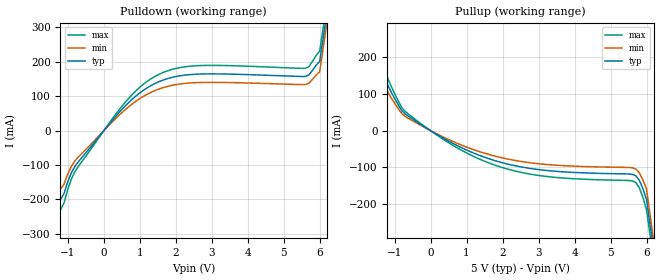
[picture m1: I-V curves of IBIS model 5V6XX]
[IBIS Ver]   2.1
[File name]   55202_5.ibs
[File Rev]   2.0
[Date]   7/20/01
[Source]   ICS MicroClock Applications Engineering 2
[Disclaimer] This information is for modeling purposes only, and is
(C) Copyright Integrated Circuit Systems, Inc. 1997-2001
   All rights reserved
ICS hereby grants the user of this IBIS model a non-exclusive,
nontransferable license to use this IBIS model under the following terms.
Before using this IBIS model, the user should read this license.
If the user does not accept these terms,  the IBIS model should be
returned to ICS within 30 days.
   The user is granted this license only to use the IBIS model and
is not granted rights to sell, load, rent, lease or license the IBIS
model in whole or in part, or in modified form to anyone other than
user. User may modify the IBIS model to suit its specific
applications but rights to derivative works and such modifications
shall belong to ICS.
   This IBIS model is provided on an "AS IS" basis and ICS makes
absolutely no warranty with respect to the information contained
herein. ICS DISCLAIMS AND CUSTOMER WAIVES ALL WARRANTIES, EXPRESS
OR IMPLIED, INCLUDING WARRANTIES OF MERCHANTABILITY OR FITNESS FOR
A PARTICULAR PURPOSE. The entire risk as to quality and performance
is with the Customer. ACCORDINGLY, IN NO EVENT SHALL THE COMPANY BE
LIABLE FOR ANY DAMAGES, WHETHER IN CONTRACT OR TORT,INCLUDING ANY
LOST PROFITS OR OTHER INCIDENTAL, CONSEQUENTIAL, EXEMPLARY, OR
PUNITIVE DAMAGES ARISING OUT OF THE USE OR APPLICATION OF THE IBIS
model provided in this package. Further, ICS reserves the right to
make changes without notice to any product herein to improve
reliability, function, or design. ICS does not convey any license
under patent rights or any other intellectual property rights,
including those of third parties.
   ICS is not obligated to provide maintenance or support
for the licensed IBIS model.
[Component]   ICS552-02
[Manufacturer] Integrated Circuit Systems Inc.
[Package]
|   typ   min   max
R_pkg   40m   35m   45m
L_pkg   1.65nH   1.35nH   1.95nH
C_pkg   0.24pF   0.14pF   0.34pF
[pin]   signal_name   model_name   R_pin   L_pin   C_pin
   3   Q0   5V6XX
   4   Q1   5V6XX
   5   Q2   5V6XX
   6   Q3   5V6XX
 11   Q4   5V6XX
 12   Q5   5V6XX
 13   Q6   5V6XX
 14   Q7   5V6XX
| Models and submodels in the file (1): 5V6XX (Output)
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|   ICS552-02 5V Clock Drive Model
| This model is suitable for all output pins on the
| ICS552-02
[Model]   5V6XX
Model_type   Output
Polarity   Non-Inverting
|   typ   min   max
C_comp   5pF   4pF   6pF
|   typ   min   max
[Voltage range]  5.0V   4.5V   5.5V
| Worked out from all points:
|   slope of the pulldown table from 0 to 0.75 V, typ, clamps not added: 8.57 ohm
|   slope of the pullup table from 0 to 0.75 V, typ, clamps not added: 18.2 ohm
[pulldown]
|Voltage I (typ)   I (min)   I (max)
-5V       -3A        -3A        -3A
-1.2V     -200mA     -170mA     -230mA
-1.1V     -182.6mA   -155.2mA   -210mA
-900mV    -123.3mA   -104.8mA   -141.8mA
-800mV    -103.9mA   -88.33mA   -119.5mA
300mV     36.86mA    31.33mA    42.39mA
1V        108.8mA    92.45mA    125.1mA
1.7V      148.1mA    125.9mA    170.3mA
2.8V      164.1mA    139.5mA    188.7mA
5.6V      156.9mA    133.3mA    180.4mA
6V        200.3mA    170.3mA    230.4mA
10V       3A         3A         3A
[pullup]
|Voltage I (typ)   I (min)   I (max)
-5V       3A         3A         3A
-1.4V     185.7mA    157.9mA    213.6mA
-1.3V     150.3mA    127.8mA    172.9mA
-1.1V     105.9mA    90.04mA    121.8mA
-700mV    44.96mA    38.22mA    51.71mA
500mV     -28.73mA   -24.42mA   -33.04mA
1.6V      -76.04mA   -64.63mA   -87.44mA
3.1V      -107.5mA   -91.34mA   -123.6mA
5.6V      -119.2mA   -101.3mA   -137.1mA
5.8V      -135.5mA   -115.2mA   -155.9mA
6V        -188mA     -159.8mA   -216.2mA
10V       -3A        -3A        -3A
[Ramp]
|   typ   min   max
dV/dt_r   2.52/0.34n   2.34/0.37n   2.65/0.31n
dV/dt_f   2.59/0.32n   2.46/0.35n   2.72/0.29n
